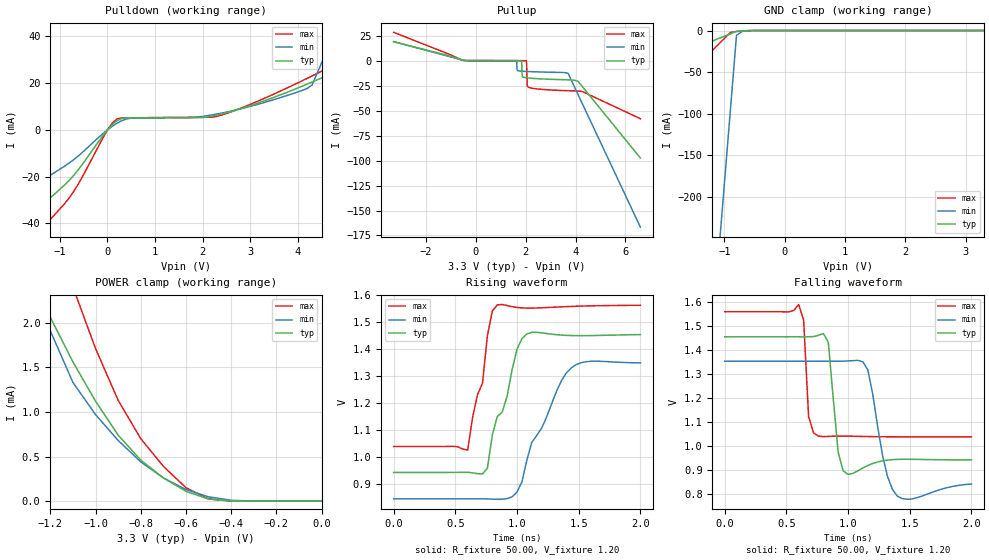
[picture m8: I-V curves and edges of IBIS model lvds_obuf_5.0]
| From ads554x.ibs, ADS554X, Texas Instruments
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|   Model lvds_obuf_5.0
[Model]   lvds_obuf_5.0
Model_type   3-state
Polarity   Non-Inverting
Enable   Active-High
Vmeas =   1.2000V
Cref =   5.0000pF
Rref = 50.0000
Vref =   1.2000V
C_comp   2.13pF   1.93pF   2.33pF
[Temperature Range]   27.00   125   -40.00
[Voltage Range]   3.30V   3.00V   3.60V
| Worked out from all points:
|   slope of the pulldown table from 0 to 0.495 V, typ, clamps not added: 96.1 ohm
|   GND clamp passes 1 mA (typ) near -0.79 V on its own axis
|   POWER clamp passes 1 mA (typ) near -0.97 V on its own axis
|   rising waveform, R_fixture 50.00, V_fixture 1.20: 20-80 % time 187ps typ, 266ps min, 124ps max; typ from 0.944 V to 1.46 V
|   falling waveform, R_fixture 50.00, V_fixture 1.20: 20-80 % time 53.7ps typ, 101ps min, 31.2ps max; typ from 1.46 V to 0.944 V
[Pulldown]
| voltage   I(typ)   I(min)   I(max)
-3.3V     -67.53mA   -46.53mA   -85.59mA
-2.1V     -45.57mA   -31.05mA   -58.59mA
-1.5V     -34.59mA   -23.31mA   -45.09mA
-800mV    -21.57mA   -14.17mA   -29.04mA
200mV     3.89mA     2.77mA     4.62mA
2.4V      6.73mA     7.11mA     6.29mA
4.3V      20.39mA    19.15mA    22.97mA
4.7V      24.03mA    38.05mA    27mA
4.9V      30.27mA    47.5mA     29.04mA
5.1V      49.2mA     56.95mA    31.28mA
5.5V      87.06mA    75.85mA    61.91mA
6.6V      191.2mA    127.8mA    180.5mA
[Pullup]
| voltage   I(typ)   I(min)   I(max)
|   100   100
-3.3V     18.97mA    19.11mA    28.41mA
-500mV    370uA      560uA      340uA
1.62V     34.26uA    17.49uA    55.86uA
1.66V     32.44uA    -9.441mA   53.53uA
1.82V     23.2uA     -10.47mA   44.15uA
1.86V     -15.23mA   -10.54mA   41.79uA
2.02V     -17.09mA   -10.77mA   11.86uA
2.06V     -17.2mA    -10.82mA   -24.35mA
2.1V      -17.3mA    -10.87mA   -26.46mA
3.7V      -19.14mA   -12.66mA   -30.03mA
4.1V      -20.66mA   -33.9mA    -30.35mA
6.6V      -97.41mA   -166.7mA   -58.09mA
[GND_clamp]
| voltage   I(typ)   I(min)   I(max)
-3.3V     -73.53mA   -2.228A    -176.7mA
-1.1V     -9.73mA    -272.6mA   -16.77mA
-1V       -6.83mA    -183.7mA   -9.5mA
-900mV    -3.93mA    -94.8mA    -2.23mA
-800mV    -1.03mA    -5.92mA    -1.19mA
-700mV    -450uA     -730uA     -490uA
3.3V      44.64pA    1.08uA     37.43pA
[POWER_clamp]
| voltage   I(typ)   I(min)   I(max)
-3.3V     247.8mA    491.9mA    558.7mA
-1.3V     2.62mA     3.21mA     3.99mA
-1.2V     2.06mA     1.91mA     3.16mA
-1.1V     1.56mA     1.33mA     2.4mA
-1V       1.12mA     970uA      1.71mA
-900mV    740uA      680uA      1.13mA
-800mV    460uA      440uA      700uA
-700mV    260uA      260uA      390uA
-600mV    110uA      130uA      150uA
-500mV    23.34uA    48.47uA    24.97uA
-400mV    2uA        9.55uA     1.31uA
0V        44.64pA    500pA      43.31pA
[Ramp]
| variable   typ   min   max
dV/dt_r   1.84/71.06p   1.61/0.12n   2.05/47.45p
dV/dt_f   1.81/0.19n   1.61/0.15n   1.91/0.31n
R_load = 1.00k
[Rising Waveform]
R_fixture = 50.00
V_fixture = 1.20
V_fixture_min = 1.10
V_fixture_max = 1.30
| time   V(typ)   V(min)   V(max)
0s        943.8mV    845.8mV    1.04V
600ps     944.4mV    845.9mV    1.027V
720ps     938mV      845.8mV    1.274V
760ps     960mV      845.5mV    1.451V
840ps     1.151V     844mV      1.565V
920ps     1.227V     846.8mV    1.563V
1ns       1.401V     871.1mV    1.556V
1.08ns    1.458V     989.9mV    1.553V
1.44ns    1.452V     1.332V     1.559V
2ns       1.455V     1.35V      1.564V
[Falling Waveform]
R_fixture = 50.00
V_fixture = 1.20
V_fixture_min = 1.10
V_fixture_max = 1.30
| time   V(typ)   V(min)   V(max)
0s        1.456V     1.355V     1.561V
600ps     1.456V     1.355V     1.591V
640ps     1.456V     1.355V     1.526V
680ps     1.457V     1.355V     1.125V
760ps     1.462V     1.355V     1.043V
840ps     1.434V     1.355V     1.042V
960ps     898.3mV    1.355V     1.043V
1.16ns    920.4mV    1.319V     1.041V
1.4ns     945.8mV    792.5mV    1.04V
2ns       943.6mV    843.3mV    1.04V
